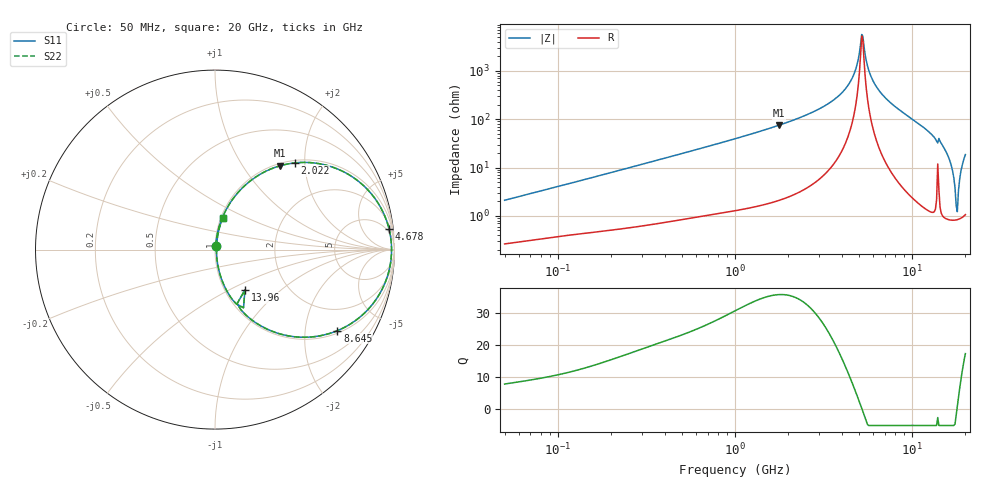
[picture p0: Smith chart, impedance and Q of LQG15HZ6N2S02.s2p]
!Murata Part Number: LQG15HZ6N2S02
!These Parameters are Measured in Series Mode Connection
!  o--[Z]--o
!Port1  Port2
!  o-------o
!Freq. Start=50[MHz] Stop=20[GHz], 401[Steps]
# Hz S RI R 50
!Freq.(Hz) S11(Real) S11(Imag) S21(Real) S21(Imag) S12(Real) S12(Imag) S22(Real) S22(Imag)
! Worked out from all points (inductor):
!   401 points, 50 MHz to 20 GHz, reference 50 ohm
!   read as one part in series: L = 6.58 nH near 51.52 MHz
!   highest Q = 35.9 at 1.767 GHz (marker M1), where L = 6.75 nH
!   self-resonance near 5.195 GHz
!   S11 on the Smith chart (normalised r, x): 50 MHz: 1.01, +0.04; 2.022 GHz: 1.05, +1.78; 4.678 GHz: 3, +16; 8.645 GHz: 1.08, -2.96; 13.96 GHz: 1.24, -0.60; 20 GHz: 1.02, +0.37
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5e7  0.00306 0.0208  0.9969 -0.0208  0.9969 -0.0208  0.00306 0.0208
1.364002e8  0.0072 0.0538  0.9928 -0.0538  0.9928 -0.0538  0.0072 0.0538
3.721004e8  0.0272 0.1403  0.9728 -0.1403  0.9728 -0.1403  0.0272 0.1403
1e9  0.1426 0.3338  0.8574 -0.3338  0.8574 -0.3338  0.1426 0.3338
1.766834e9  0.3632 0.4672  0.6368 -0.4672  0.6368 -0.4672  0.3632 0.4672
2.021818e9  0.4435 0.483  0.5565 -0.483  0.5565 -0.483  0.4435 0.483
2.728004e9  0.6537 0.46  0.3463 -0.46  0.3463 -0.46  0.6537 0.46
3.850025e9  0.89 0.2864  0.11 -0.2864  0.11 -0.2864  0.89 0.2864
4.677679e9  0.97 0.1141  0.03 -0.1141  0.03 -0.1141  0.97 0.1141
5.117541e9  0.9833 0.022  0.0167 -0.022  0.0167 -0.022  0.9833 0.022
5.273168e9  0.9837 -0.00978  0.0163 0.00978  0.0163 0.00978  0.9837 -0.00978
5.598765e9  0.9783 -0.074  0.0217 0.074  0.0217 0.074  0.9783 -0.074
5.944466e9  0.9641 -0.1381  0.0359 0.1381  0.0359 0.1381  0.9641 -0.1381
7.442007e9  0.8317 -0.3547  0.1683 0.3547  0.1683 0.3547  0.8317 -0.3547
8.644534e9  0.6816 -0.4518  0.3184 0.4518  0.3184 0.4518  0.6816 -0.4518
1.115139e10  0.3679 -0.4713  0.6321 0.4713  0.6321 0.4713  0.3679 -0.4713
1.396067e10  0.1668 -0.2247  0.8332 0.2247  0.8332 0.2247  0.1668 -0.2247
1.621653e10  0.0295 -0.1438  0.9705 0.1438  0.9705 0.1438  0.0295 -0.1438
1.774144e10  0.00839 -0.014  0.9916 0.014  0.9916 0.014  0.00839 -0.014
1.828096e10  0.00946 0.0318  0.9905 -0.0318  0.9905 -0.0318  0.00946 0.0318
1.912117e10  0.0199 0.1025  0.9801 -0.1025  0.9801 -0.1025  0.0199 0.1025
2e10  0.0427 0.1756  0.9573 -0.1756  0.9573 -0.1756  0.0427 0.1756
